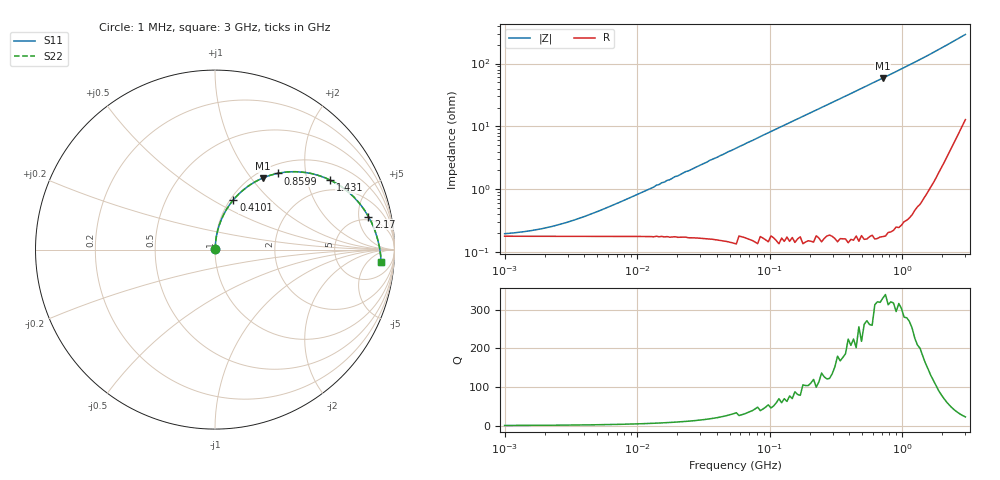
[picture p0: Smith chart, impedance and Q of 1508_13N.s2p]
# MHz S MA R 50
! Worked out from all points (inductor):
!   174 points, 1 MHz to 3 GHz, reference 50 ohm
!   read as one part in series: L = 12.9 nH near 6.669 MHz
!   highest Q = 330 at 714.6 MHz (marker M1), where L = 13.1 nH
!   S11 on the Smith chart (normalised r, x): 1 MHz: 1.00, +0.00; 410.1 MHz: 1.03, +0.63; 859.9 MHz: 1.16, +1.41; 1.431 GHz: 1.58, +2.79; 2.17 GHz: 4.29, +6.68; 3 GHz: 13, -13
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1  0.001765 25.1  0.998 -0.1  0.998 -0.1  0.001765 25.1
2.002  0.002192 43.1  0.998 -0.1  0.998 -0.1  0.002193 43.1
3.827  0.003285 60.7  0.998 -0.2  0.998 -0.2  0.003286 60.7
13.352  0.01 80.3  0.998 -0.7  0.998 -0.7  0.01 80.3
13.984  0.011 80.6  0.998 -0.7  0.998 -0.7  0.011 80.6
14.647  0.011 81.0  0.998 -0.7  0.998 -0.7  0.011 81.0
15.34  0.012 81.3  0.998 -0.8  0.998 -0.8  0.012 81.3
17.625  0.013 82.2  0.998 -0.9  0.998 -0.9  0.013 82.2
19.335  0.015 82.8  0.998 -1.0  0.998 -1.0  0.015 82.8
20.25  0.015 83.0  0.998 -1.0  0.998 -1.0  0.015 83.0
56.054  0.042 85.0  0.998 -2.8  0.998 -2.8  0.042 85.0
117.542  0.088 83.1  0.995 -5.8  0.995 -5.8  0.088 83.1
214.526  0.159 78.8  0.986 -10.6  0.986 -10.6  0.159 78.8
410.077  0.295 69.7  0.954 -20.0  0.954 -20.0  0.295 69.7
714.584  0.478 56.4  0.877 -33.4  0.877 -33.4  0.478 56.4
821.013  0.532 52.0  0.845 -37.8  0.845 -37.8  0.532 52.0
859.902  0.55 50.5  0.833 -39.3  0.833 -39.3  0.551 50.5
1135.123  0.662 40.5  0.747 -49.3  0.747 -49.3  0.662 40.5
1430.664  0.75 31.0  0.657 -58.6  0.657 -58.6  0.75 31.0
1721.606  0.812 22.9  0.576 -66.5  0.576 -66.5  0.813 22.9
2169.844  0.874 12.2  0.469 -76.8  0.469 -76.8  0.875 12.2
3000  0.928 -4.3  0.33 -91.6  0.33 -91.6  0.929 -4.3
